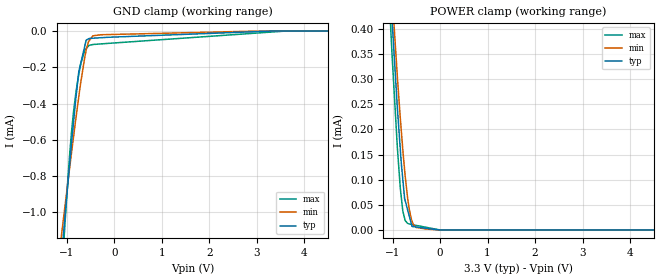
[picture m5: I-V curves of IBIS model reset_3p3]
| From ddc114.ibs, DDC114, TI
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|   reset_3p3 Model
[Model]   reset_3p3
Model_type   Input
Vinl = 0.66
Vinh = 2.64
|   typ   min   max
|   (nom PVT)   (fast PVT)   (slow PVT)
|C_comp from frequency sweep method (F=0.01MHz)
|Average
|C_comp   6.579e-13   5.497e-13   7.719e-13
|C_comp from LC tank measurement(L=1nH)
|Average
|Resonant Frequency(Hz)   5.926e+10   6.314e+10   4.494e+10
C_comp   7.220e-15   6.360e-15   1.255e-14
| Where nom  PVT is Nominal Process, 3.3V, 27C
|   Fast PVT is Strong Process,  3.6V, -40C
|   Slow PVT is Weak Process,   3V, 87C
[Model Spec]
|Subparameter   typ   min   max
Vinl   0.66   0.60   0.72
Vinh   2.64   2.4   2.88
[Voltage Range]   3.3   3   3.6
|Ambient Temperature   25   85   -40
|Junction Temperature
[Temperature Range]   27   87   -40
[Power Clamp Reference]   3.3   3   3.6
[GND Clamp Reference]   0   0   0
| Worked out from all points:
|   GND clamp passes 1 mA (typ) near -1.03 V on its own axis
|   POWER clamp passes 1 mA (typ) near -1.34 V on its own axis
[GND Clamp]
|   Voltage   I(typ)   I(min)   I(max)
-3.3V     -8.298mA   -6.122mA   -11.81mA
-1.175V   -1.448mA   -1.271mA   -1.662mA
-1.08V    -1.158mA   -1.062mA   -1.241mA
-1.02V    -973.9uA   -931.4uA   -996.3uA
-932.4mV  -717.9uA   -743.9uA   -663.1uA
-856.8mV  -504.8uA   -585.8uA   -446.6uA
-759.6mV  -257.8uA   -390.3uA   -259.7uA
-702mV    -175.6uA   -280.6uA   -179.1uA
-590.7mV  -50.54uA   -106.1uA   -97.21uA
-447mV    -39.3uA    -26.25uA   -74.09uA
3.6V      0A         0A         0A
6.6V      0A         0A         0A
[POWER Clamp]
|   Voltage   I(typ)   I(min)   I(max)
-3.3V     4.89mA     4.568mA    5.322mA
-1.145V   647.7uA    681.7uA    605.4uA
-1.026V   443.9uA    493.1uA    379.5uA
-1.004V   409.6uA    461uA      339.8uA
-896.4mV  240.7uA    302.8uA    161.7uA
-835.2mV  159.6uA    221.9uA    82.55uA
-784.8mV  102.3uA    161.3uA    38.96uA
-745.8mV  62.84uA    120.2uA    23.27uA
-681mV    39.69uA    62.78uA    13.18uA
-580.8mV  6.937uA    15.55uA    10.64uA
-33.83fV  0A         0A         0A
6.6V      0A         0A         0A
